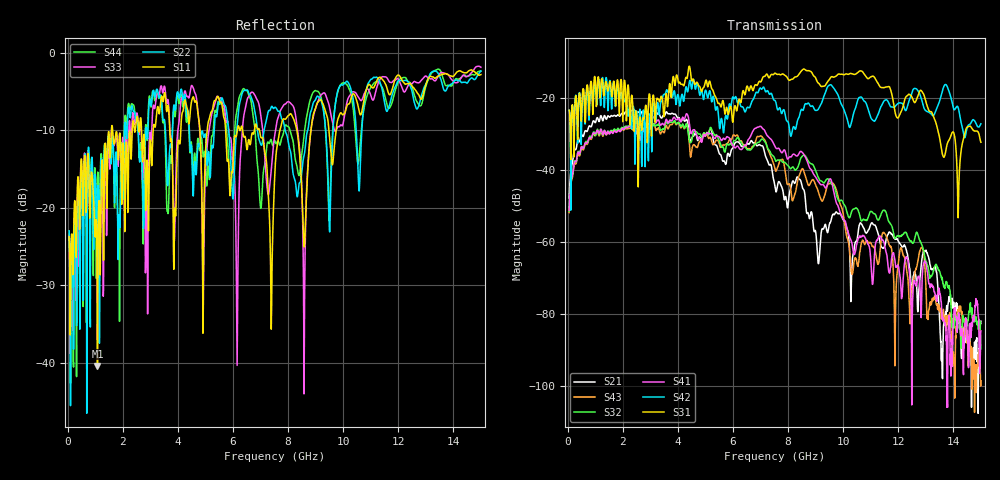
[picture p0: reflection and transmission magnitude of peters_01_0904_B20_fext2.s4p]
# MHZ S RI R 50.00
! FREQ  S11  S12  S13  S14
!  S21  S22  S23  S24
!  S31  S32  S33  S34
!  S41  S42  S43  S44
!  REAL  IMAG  REAL  IMAG  REAL  IMAG  REAL  IMAG
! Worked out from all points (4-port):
!   1496 points, 50 MHz to 15 GHz, reference 50 ohm
!   strongest paths, dB at 50 MHz, 3.79 GHz, 7.53 GHz, 11.27 GHz, 15 GHz:
!     S31: -23.3, -16.5, -13.0, -15.9, -32.3
!     S42: -23.3, -19.6, -20.7, -24.5, -27.1
!     S41: -51.2, -26.2, -33.5, -59.0, -84.8
!     S32: -51.5, -26.7, -37.2, -53.9, -89.7
!     S43: -51.8, -27.3, -39.9, -66.2, -98.6
!     S21: -47.8, -24.2, -45.0, -57.7, -82.0
!   lowest |S11| = -40.4 dB at 1.08 GHz (marker M1), VSWR 1.02, Z = 50.5 + j0.829 ohm
!   |S11| at or under -10 dB: start of sweep to 1.585 GHz; 1.631 GHz to 2.34 GHz (709.4 MHz wide, 35.7 % of centre); 6.962 GHz to 7.703 GHz (741.1 MHz wide, 10.1 % of centre)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
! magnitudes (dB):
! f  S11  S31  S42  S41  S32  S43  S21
! 50 MHz  -23.7  -23.3  -23.3  -51.2  -51.5  -51.8  -47.8
! 1.08 GHz  -40.4  -15.7  -18.9  -29.0  -28.6  -29.3  -25.4
! 6.15 GHz  -10.1  -23.1  -21.0  -33.3  -31.0  -30.2  -32.2
! 7.01 GHz  -10.9  -15.5  -17.3  -27.8  -31.6  -30.5  -33.2
! 8.59 GHz  -25.0  -11.9  -22.2  -35.9  -35.8  -40.8  -45.9
! 9.22 GHz  -6.2  -16.8  -21.3  -44.1  -43.1  -48.6  -56.6
! 15 GHz  -2.8  -32.3  -27.1  -84.8  -89.7  -98.6  -82.0
